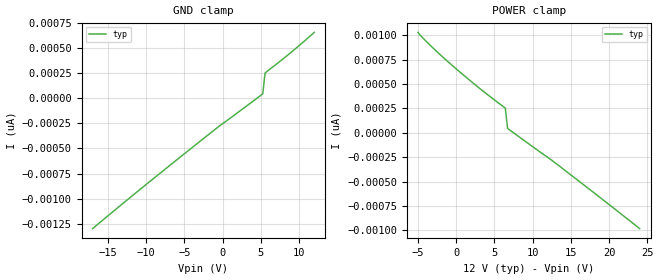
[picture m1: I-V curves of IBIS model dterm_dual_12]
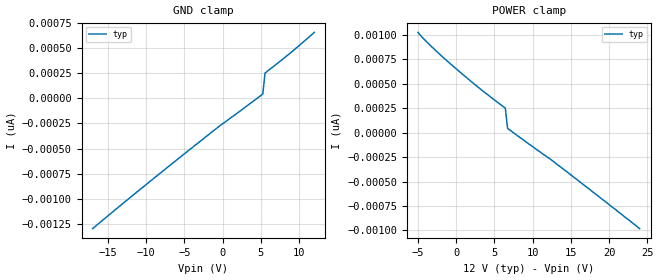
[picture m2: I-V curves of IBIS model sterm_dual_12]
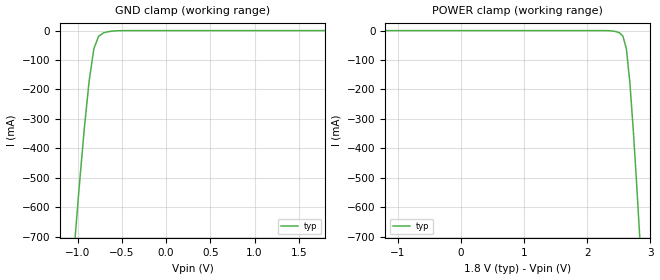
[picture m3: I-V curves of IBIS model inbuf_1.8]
|Texas Instruments Incorporated
|tmux4827, 2 Data Lane 2:1 +/-12V Precision mux
[IBIS Ver]   4.1
[File name]   tmux4827.ibs
[Date]   05/30/23
[File Rev]   1.0
[Source]
| Texas Instruments Incorporated.
| ASC-INT-MPD
| 12500 TI Blvd
| Dallas, TX - 75243
[Notes]   Revision History:
| Rev 1.0: 05/30/23
| - Initial version of the model
| - Model generated from simulations in SPECTRE
| - C_comp although listed in numerical order of value are
|   obtained from varying PVT conditions. For PVT conditions for
|   each specific value refer the buffer description under
|   respective [Model]. IBIS model user is responsible for using
|   appropriate C_comp to simulate for Signal Integrity.
[Disclaimer]
| This model is designed as an aid for customers of Texas Instruments.
| TI and its licensors and suppliers make no warranties, either expressed
| or implied, with respect to this  model, including the warranties of
| merchantability or fitness for a particular purpose. The model is
| provided solely on an "as is" basis. The entire risk as to its quality
| and performance is with the customer.
| This model is subject to change without notice. Texas Instruments
| Incorporated is not responsible for updating this model.
[Copyright]
(C) Copyright 2023 Texas Instruments Incorporated.All rights reserved.
|  Component TMUX4827YBH 9-pin - YBH package
|  Part # TMUX4827YBH
[Component]   TMUX4827YBH
[Manufacturer]  TI
[Package]
|   typ   min   max
R_pkg   0   NA   NA
L_pkg   0   NA   NA
C_pkg   0   NA   NA
[Pin]   signal_name   model_name
   A1   S1A   sterm
   A2   SEL   inbuf
   A3   S2A   sterm
   B1   D1   dterm
   B2   GND   gnd
   B3   D2   dterm
   C1   S1B   sterm
   C2   VDD   power
   C3   S2B   sterm
[Series Switch Groups]
On 1 /
On 2 /
Off 1 /
[Series Pin Mapping]  pin_2 model_name function_table_group
  A1   B1   switch_dual_12   1
  A3   B3   switch_dual_12   1
  C1   B1   switch_dual_12   2
  C3   B3   switch_dual_12   2
[Model Selector] dterm
dterm_dual_12 Use for operation at +/-12V
[Model Selector] sterm
sterm_dual_12 Use for operation at +/-12V
[Model Selector] inbuf
inbuf_1.8 Use for operation at 1V
inbuf_5.5 Use for operation at 5V
inbuf_3.3 Use for operation at 3V
| switch_dual_12
[Model]   switch_dual_12
Model_type   Series_switch
|   typ   min   max
C_comp   4.014581e-11   NA   NA
[Voltage Range]   12   NA   NA
[Power Clamp Reference]   12   NA   NA
[Temperature Range]   27   NA   NA
[On]
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[Off]
|   typ   min   max
[R Series]   10G   NA   NA
| inbuf_5.5
[Model]   inbuf_5.5
Model_type   Input
Vinl = 0.8
Vinh = 1.2
|   typ   min   max
C_comp   2.533030e-12   NA   NA
[Voltage Range]   5.5   NA   NA
[Temperature Range]   27   NA   NA
[Power Clamp Reference]   5.5   NA   NA
[GND Clamp Reference]   0   NA   NA
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| Models and submodels in the file (6): dterm_dual_12 (Terminator), switch_dual_12 (Series_switch), sterm_dual_12 (Terminator), inbuf_1.8 (Input), inbuf_5.5 (Input), inbuf_3.3 (Input)
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| dterm_dual_12
[Model]   dterm_dual_12
Model_type   Terminator
|   typ   min   max
C_comp   4.014581e-11   NA   NA
[Voltage Range]   12   NA   NA
[Temperature Range]   27   NA   NA
[Power Clamp Reference]   12   NA   NA
[GND Clamp Reference]   0   NA   NA
[GND Clamp]
|   Voltage   I(typ)   I(min)   I(max)
-17V      -1.299nA   NA         NA
-10.56V   -893.5pA   NA         NA
-2.061V   -375.7pA   NA         NA
5.263V    43.26pA    NA         NA
5.556V    250pA      NA         NA
8.778V    444.4pA    NA         NA
12V       654.5pA    NA         NA
[POWER Clamp]
|   Voltage   I(typ)   I(min)   I(max)
-5V       1.028nA    NA         NA
-3.535V   905.7pA    NA         NA
-606.1mV  695.1pA    NA         NA
2.909V    463.9pA    NA         NA
6.424V    251.5pA    NA         NA
6.717V    44.84pA    NA         NA
12.58V    -286.6pA   NA         NA
24V       -982.6pA   NA         NA
| sterm_dual_12
[Model]   sterm_dual_12
Model_type   Terminator
|   typ   min   max
C_comp   4.014581e-11   NA   NA
[Voltage Range]   12   NA   NA
[Temperature Range]   27   NA   NA
[Power Clamp Reference]   12   NA   NA
[GND Clamp Reference]   0   NA   NA
[GND Clamp]
|   Voltage   I(typ)   I(min)   I(max)
-17V      -1.297nA   NA         NA
-10.56V   -892.6pA   NA         NA
-2.061V   -375.6pA   NA         NA
5.263V    42.82pA    NA         NA
5.556V    250.7pA    NA         NA
8.778V    445.6pA    NA         NA
12V       655.8pA    NA         NA
[POWER Clamp]
|   Voltage   I(typ)   I(min)   I(max)
-5V       1.027nA    NA         NA
-3.535V   904.6pA    NA         NA
-606.1mV  694.2pA    NA         NA
2.909V    463.3pA    NA         NA
6.424V    251.1pA    NA         NA
6.717V    44.54pA    NA         NA
12.58V    -286.5pA   NA         NA
24V       -981.9pA   NA         NA
| inbuf_1.8
[Model]   inbuf_1.8
Model_type   Input
Vinl = 0.8
Vinh = 1.2
|   typ   min   max
C_comp   2.533030e-12   NA   NA
[Voltage Range]   1.8   NA   NA
[Temperature Range]   27   NA   NA
[Power Clamp Reference]   1.8   NA   NA
[GND Clamp Reference]   0   NA   NA
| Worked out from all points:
|   GND clamp passes 1 mA (typ) near -0.57 V on its own axis
[GND Clamp]
|   Voltage   I(typ)   I(min)   I(max)
-3.6V     -6.939A    NA         NA
-1.036V   -723.3mA   NA         NA
-981.8mV  -522.1mA   NA         NA
-927.3mV  -334.7mA   NA         NA
-872.7mV  -173.2mA   NA         NA
-818.2mV  -61.21mA   NA         NA
-763.6mV  -18.79mA   NA         NA
-709.1mV  -7.682mA   NA         NA
-545.5mV  -484.8uA   NA         NA
1.8V      51.95pA    NA         NA
[POWER Clamp]
|   Voltage   I(typ)   I(min)   I(max)
-1.8V     112.6pA    NA         NA
2.291V    -112.4uA   NA         NA
2.4V      -1.496mA   NA         NA
2.509V    -7.682mA   NA         NA
2.564V    -18.79mA   NA         NA
2.618V    -61.21mA   NA         NA
2.673V    -173.2mA   NA         NA
2.727V    -334.7mA   NA         NA
2.782V    -522.1mA   NA         NA
2.836V    -723.3mA   NA         NA
3.6V      -3.282A    NA         NA
